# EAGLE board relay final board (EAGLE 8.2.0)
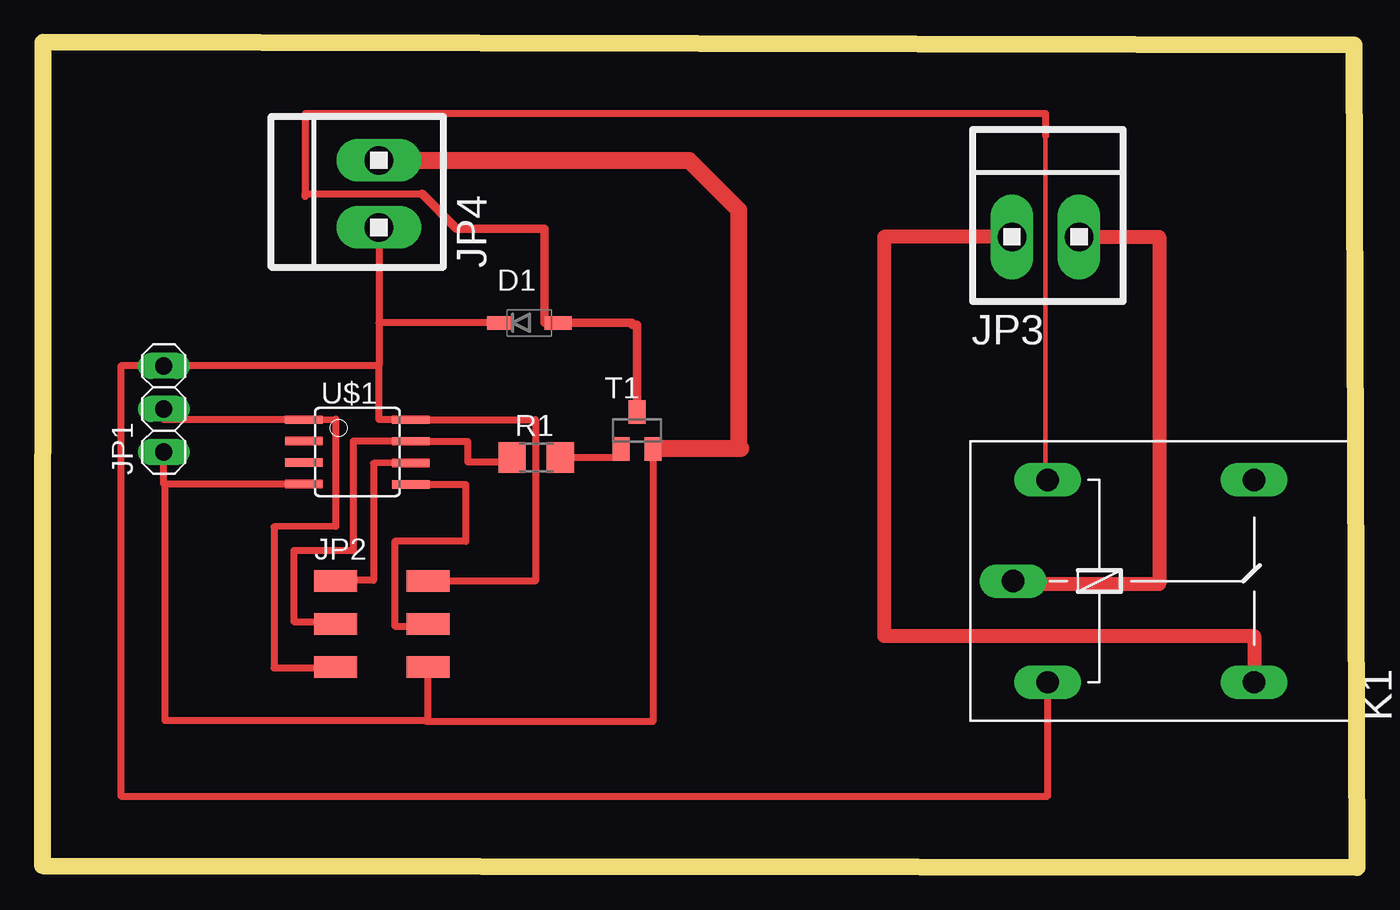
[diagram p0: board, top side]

Size 77.65 x 48.7 mm. Coordinates in mm from the lower left corner, seen from the top.
Outline: 0,0.1 77.65,0 77.48,48.54 0.03,48.7 0,0.1
Copper layers (1*16): Top 0.035mm / dielectric 1.5mm / Bottom 0.035mm
Design rules "default": minimum track width 10mil, minimum drill 24mil, track to track 8mil, track to pad 8mil, pad to pad 8mil, via to via 8mil, smd to smd 8mil, copper to edge 40mil, drill to drill 8mil, minimum pad ring 10mil, minimum via ring 8mil, stop-mask expansion 4mil, vias tented up to drill 0mil, thermal gap 10mil

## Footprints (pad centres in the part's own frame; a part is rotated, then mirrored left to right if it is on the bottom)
SOD123 = smd 1.6 x 0.8: ANODE 1.7,0; CATHODE -1.7,0
1X03 = drill 1.016 long: 1 -2.54,0; 2 0,0; 3 2.54,0
2X03SMD = smd 2.54 x 1.27: 1 -2.54,2.54; 2 2.92,2.54; 3 -2.54,0; 4 2.92,0; 5 -2.54,-2.54; 6 2.92,-2.54
1X2MTA = drill 1.676 long: 1 1.981,0; 2 -1.981,0
G5LE = drill 1.321 long: 1 -7.493,-5.969; 2 -7.493,5.969; O 4.699,5.969; P -9.525,0; S 4.699,-5.969
R1206 = smd 1.6 x 1.803: 1 -1.422,0; 2 1.422,0
SOT23 = smd 1 x 1.4: 1 -0.95,-1.1; 2 0.95,-1.1; 3 0,1.1
SOIC8 = smd 0.5 x 2.2: 1 -1.905,-3.154; 2 -0.645,-3.154; 3 0.625,-3.154; 4 1.895,-3.154; 5 1.905,3.154; 6 0.635,3.154; 7 -0.635,3.154; 8 -1.905,3.154

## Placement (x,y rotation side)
D1  [SOD123]  28.76,32.14 0 top
JP1  [1X03]  7.18,27.06 90 top
JP2  [2X03SMD]  19.88,14.36 0 top
JP3  [1X2MTA]  59.25,37.22 0 top
JP4  [1X2MTA]  19.88,39.76 90 top
K1  G5L  [G5LE]  66.87,16.9 0 top
R1  [R1206]  29.17,24.2 0 top
T1  BC846  [SOT23]  35.11,25.79 0 top
U$1  ATTINY45SI  [SOIC8]  18.61,24.52 270 top

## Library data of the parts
D1 JP2 R1 U$1 = fab
JP1 = pinhead
JP3 JP4 = con-amp
K1 = relay; OC_FARNELL: unknown; OC_NEWARK: unknown
T1 = transistor

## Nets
N$1: JP1.1 JP2.6 JP4.1 T1.2 U$1.4
N$2: D1.CATHODE JP1.3 JP2.2 JP4.2 K1.1 U$1.8
N$3: JP1.2 JP2.5 U$1.1
N$4: JP2.4 U$1.5
N$5: JP2.3 R1.1 U$1.7
N$6: JP2.1 U$1.6
N$7: JP3.1 K1.P
N$9: D1.ANODE K1.2 T1.3
N$10: R1.2 T1.1
N$11: JP3.2 K1.S

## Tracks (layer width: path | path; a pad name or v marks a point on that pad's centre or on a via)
N$1
  Top 0.254: 15.43,22.62 U$1.4 | 35.75,24.52 T1.2 36.39,25.16
  Top 0.406: 15.43,22.62 7.23,22.62 | JP1.1 7.18,22.62 7.23,22.62 | 36.39,25.16 36.06,25.16 | 23.11,11.82 JP2.6 22.79,8.67 22.68,8.67 | 36.06,24.62 T1.2 | 7.23,22.62 7.23,8.67 22.68,8.67 | 36,25.16 36.06,25.16 | 36.06,25.16 36.06,24.48 36.06,8.6 22.68,8.6 22.68,8.67
  Top 1.016: JP4.1 38.19,41.74 41.12,38.82 41.12,24.84 41.24,24.73 36.31,24.73 36.06,24.48
N$2
  Top 0.254: 21.14,26.43 U$1.8
  Top 0.406: 21.14,26.43 19.88,26.43 19.88,29.6 | 19.88,29.6 JP1.3 4.64,29.6 4.64,4.2 59.37,4.2 K1.1 | D1.CATHODE 19.88,32.14 | 19.88,32.14 19.88,29.6 | JP4.2 19.88,32.14 | U$1.8 29.13,26.43 29.13,16.91 JP2.2
N$3
  Top 0.254: 15.43,26.43 U$1.1
  Top 0.406: 15.43,26.43 7.18,26.43 JP1.2 | U$1.1 17.33,26.47 17.33,20.14 13.69,20.09 13.69,11.77 17.34,11.77 JP2.5
N$4
  Top 0.406: 22.79,14.47 JP2.4 22.79,14.24 20.81,14.24 20.81,19.25 25,19.25 25,22.62 U$1.5
N$5
  Top 0.406: R1.1 27.75,23.95 25.13,23.95 25.13,25.16 U$1.7 18.36,25.16 18.36,18.7 14.86,18.7 14.86,14.51 17.34,14.51 JP2.3
N$6
  Top 0.406: U$1.6 19.55,23.84 19.55,16.95 17.34,16.95 JP2.1
N$7
  Top 0.406: 57.34,16.72 K1.P
  Top 0.813: JP3.1 65.97,37.22 65.97,16.72 57.34,16.72
N$9
  Top 0.254: 59.25,43.57 59.25,43.17 59.25,23.25 K1.2
  Top 0.406: 22.42,39.76 15.5,39.76 15.5,39.62 15.55,39.62 15.55,44.51 59.25,44.51 59.25,43.17
  Top 0.508: 22.42,39.76 24.47,37.7 29.65,37.7 29.65,32.14 D1.ANODE 34.83,32.14 34.83,32.02 35.11,32.02 T1.3
N$10
  Top 0.254: 33.84,24.52 T1.1
  Top 0.406: T1.1 34.17,24.2 R1.2
N$11
  Top 0.813: JP3.2 49.72,37.22 49.72,13.67 71.56,13.67 K1.S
